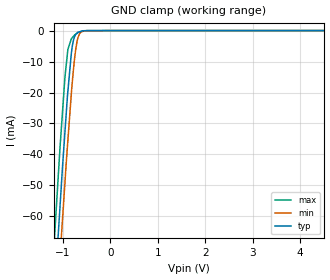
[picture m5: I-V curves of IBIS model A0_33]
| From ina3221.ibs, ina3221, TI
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|   A0 input model
[Model]   A0_33
Model_type   Input
Vinl = 0.99   |min, GND -0.5 V
Vinh = 2.31   |max. V+ 6 V
|   typ   min   max
|   (nom PVT)   (Fast PVT)   (slow PVT)
C_comp   5.755E-13   5.651E-13   6.167E-13
| Where   nom PVT is Nominal Process, 3.3V, 25C
|   Fast PVT is Strong Process, 3.6V, -40C
|   Slow PVT is Weak Process, 3.0V, 85C
|C_comp - from L-C Tank method, L = 1nH, peak frequency
[Model Spec]
| variable   typ   min   max
Vinl   0.99   0.9   1.08
Vinh   2.31   2.1   2.52
|Vinl = 0.3 x V+, Vinh = 0.7 x V+
[Voltage Range]   3.3   3   3.6
|Ambient Temperature Range   27   85   -40
[Temperature Range]   30   88   -40
[Power Clamp Reference]   3.3   3   3.6
[GND Clamp Reference]   0   0   0
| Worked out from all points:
|   GND clamp passes 1 mA (typ) near -0.71 V on its own axis
[GND Clamp]
|   Voltage   I(typ)   I(min)   I(max)
-3.3V     -649.7mA   -656.5mA   -642.6mA
-1.178V   -84.67mA   -101.3mA   -66.35mA
-1.075V   -59.75mA   -76.11mA   -40.8mA
-1.064V   -56.98mA   -73.39mA   -37.96mA
-1.016V   -45.31mA   -62.27mA   -27.45mA
-958.6mV  -32.61mA   -48.92mA   -14.93mA
-897.4mV  -19.64mA   -35.49mA   -6.081mA
-803.9mV  -5.045mA   -16.67mA   -2.273mA
-731.9mV  -1.28mA    -6.1mA     -1.161mA
-683.6mV  -535.5uA   -2.309mA   -623.7uA
-571.3mV  -63.02uA   -161.1uA   -123.6uA
6.59V     0A         0A         0A
[POWER Clamp]
|   SCR cell for ESD function. Effects occurr above VDD x 2
|   Voltage   I(typ)   I(min)   I(max)
-3.3V     0A         0A         0A
0V        0A         0A         0A
6.6V      0A         0A         0A
